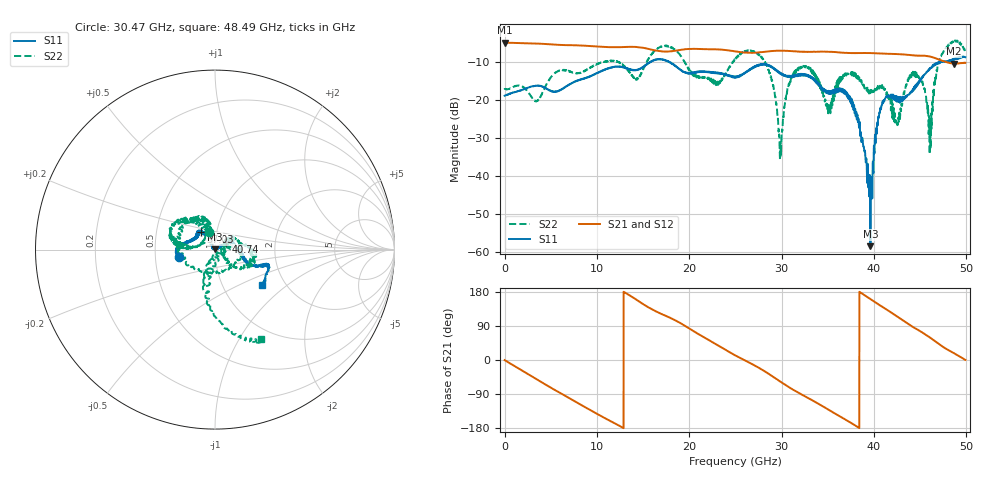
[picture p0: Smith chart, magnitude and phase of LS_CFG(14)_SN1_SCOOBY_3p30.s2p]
!Keysight Technologies,N5245B,MY58422026,A.13.80.08
!Date: Thursday, March 19, 2020 23:31:03
!Correction: S11(Full 2 Port(1,2))
!S21(Full 2 Port(1,2))
!S12(Full 2 Port(1,2))
!S22(Full 2 Port(1,2))
!S2P File: Measurements: S11, S21, S12, S22:
# Hz S DB R 50.0
!freq dBS11 angS11 dBS21 angS21 dBS12 angS12 dBS22 angS22
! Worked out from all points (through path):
!   4991 points, 10 MHz to 49.91 GHz, reference 50 ohm
!   highest |S21| = -5.02 dB at 20 MHz (marker M1); lowest = -10.5 dB at 48.67 GHz (marker M2)
!   group delay of S21, straight-line fit = 39.6 ps
!   lowest |S11| = -58.4 dB at 39.62 GHz (marker M3), VSWR 1.00, Z = 49.9 + j0.0884 ohm
!   |S11| at or under -10 dB: start of sweep to 15.82 GHz; 17.79 GHz to 47.22 GHz (29.43 GHz wide, 90.5 % of centre); 47.24198 GHz to 47.31273 GHz (70.76 MHz wide, 0.15 % of centre)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
!   |S22| runs from -35.8 to -4.4 dB; largest |S21 - S12| = 0.0053
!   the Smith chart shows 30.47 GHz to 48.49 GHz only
!   S11 on the Smith chart (normalised r, x): 30.47 GHz: 0.67, -0.06; 37.03 GHz: 0.84, +0.17; 40.74 GHz: 1.13, +0.10; 48.49 GHz: 1.52, -0.67
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1e7  -18.93 -1.7  -5.02 -0.3  -5.01 -0.3  -16.94 0.3
2e7  -18.90 -0.7  -5.02 -0.4  -5.01 -0.4  -17.10 -0.5
8.33e9  -14.69 -73.7  -5.77 -119.0  -5.77 -118.9  -12.82 -79.1
1.665e10  -9.38 -125.0  -7.20 125.4  -7.19 125.4  -6.43 -161.8
2.299e10  -13.07 -141.8  -6.77 40.4  -6.77 40.4  -15.97 -173.6
2.496e10  -14.07 -139.2  -7.28 12.5  -7.26 12.6  -9.47 -178.1
2.819e10  -10.81 -159.1  -7.41 -30.1  -7.41 -30.0  -10.20 -97.1
2.987e10  -13.23 -169.2  -7.14 -57.0  -7.13 -56.9  -31.80 16.2
3.047e10  -13.89 -168.6  -7.16 -66.6  -7.16 -66.4  -19.69 110.1
3.328e10  -14.11 171.8  -7.42 -105.9  -7.41 -105.6  -12.44 169.7
3.507e10  -17.92 144.6  -7.38 -130.9  -7.33 -130.4  -22.42 138.6
3.703e10  -18.04 128.7  -7.71 -158.8  -7.62 -158.8  -13.09 128.5
3.962e10  -58.39 132.6  -7.75 160.7  -7.73 160.5  -17.90 -84.2
4.074e10  -22.39 34.0  -7.86 142.9  -7.87 142.7  -17.03 0.7
4.16e10  -18.80 33.1  -7.95 129.7  -7.97 129.5  -19.46 38.0
4.254e10  -19.29 31.8  -8.01 114.6  -8.03 114.4  -26.66 -7.8
4.457e10  -15.99 -10.9  -8.40 82.4  -8.42 82.3  -13.22 -8.5
4.613e10  -11.74 -20.7  -8.71 58.2  -8.72 58.1  -29.91 -39.2
4.7e10  -10.11 -15.6  -9.43 43.0  -9.44 43.0  -10.24 -97.9
4.849e10  -9.73 -37.1  -10.44 20.4  -10.46 20.4  -4.99 -62.8
4.867e10  -9.18 -39.3  -10.51 17.9  -10.52 18.0  -4.52 -56.9
4.991e10  -8.82 -38.2  -10.29 0.2  -10.31 0.1  -7.41 -24.3
